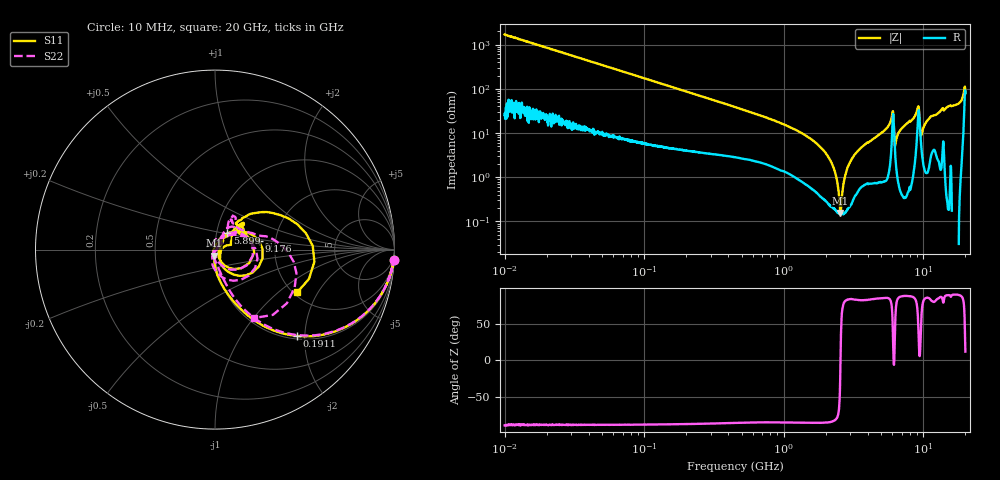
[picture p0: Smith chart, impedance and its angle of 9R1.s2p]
!Keysight Technologies,P5008B,MY61100088,A.16.20.02
!Date: Monday, November 06, 2023 16:15:06
!Correction: S11(C  2-Port  )
!S21(C  2-Port  )
!S12(C  2-Port  )
!S22(C  2-Port  )
!S2P File: Measurements: S11, S21, S12, S22:Log Frequency Sweep
# Hz S  dB  R 50
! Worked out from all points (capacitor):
!   1601 points, 10 MHz to 20 GHz, reference 50 ohm
!   read as one part in series: C = 9.38 pF near 10.39 MHz
!   lowest |Z| = 156 mohm at 2.545 GHz (marker M1)
!   series resonance near 2.548 GHz, so ESL is about 420 pH
!   S11 on the Smith chart (normalised r, x): 10 MHz: 1, -34; 191.1 MHz: 1.06, -1.83; 5.899 GHz: 1.13, +0.21; 9.176 GHz: 1.64, +0.17; 20 GHz: 2.09, -1.36
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1e7  -0.02 -3.4  -24.63 85.8  -24.62 85.8  -0.02 -3.4
3.555162e7  -0.22 -11.6  -13.96 76.8  -13.96 76.8  -0.23 -11.6
1.263918e8  -1.96 -35.4  -4.77 52.5  -4.77 52.5  -2.01 -35.5
1.910787e8  -3.56 -46.4  -2.83 41.0  -2.83 41.0  -3.68 -46.5
4.472136e8  -8.69 -66.2  -0.85 20.3  -0.85 20.4  -9.20 -65.2
1.589917e9  -20.50 -89.8  -0.13 3.1  -0.13 3.1  -22.16 -84.4
2.544636e9  -29.33 -102.5  -0.09 -1.9  -0.10 -1.9  -29.17 -105.3
3.32018e9  -42.83 156.0  -0.12 -4.6  -0.12 -4.6  -34.30 -108.9
3.995989e9  -36.54 68.7  -0.09 -6.7  -0.09 -6.7  -45.91 -34.1
4.630008e9  -36.52 72.6  -0.06 -8.9  -0.06 -8.9  -35.32 29.5
5.652411e9  -24.94 68.2  -0.11 -13.7  -0.12 -13.7  -23.92 58.9
5.899321e9  -18.85 52.6  -0.42 -17.1  -0.42 -17.1  -18.52 49.5
6.157017e9  -16.42 -45.8  -1.01 -5.7  -1.01 -5.7  -17.03 -52.6
6.738606e9  -32.96 -20.1  -0.05 -12.7  -0.05 -12.7  -39.61 159.5
8.344716e9  -24.20 54.3  -0.08 -20.2  -0.08 -20.2  -25.17 66.4
9.176444e9  -12.03 11.0  -2.00 -26.4  -2.00 -26.4  -12.83 -0.4
9.577292e9  -16.97 -59.6  -0.63 -13.7  -0.64 -13.7  -17.83 -85.1
1.063241e10  -29.64 -12.3  -0.08 -22.0  -0.08 -22.0  -56.25 84.4
1.141771e10  -22.49 18.7  -0.27 -25.1  -0.28 -25.1  -26.20 43.4
1.335558e10  -16.53 46.2  -0.20 -30.0  -0.20 -30.0  -17.43 60.9
1.862442e10  -12.04 47.1  -0.50 -52.2  -0.50 -52.2  -12.83 23.7
2e10  -5.74 -27.5  -5.71 -33.0  -5.71 -33.0  -7.15 -60.2
